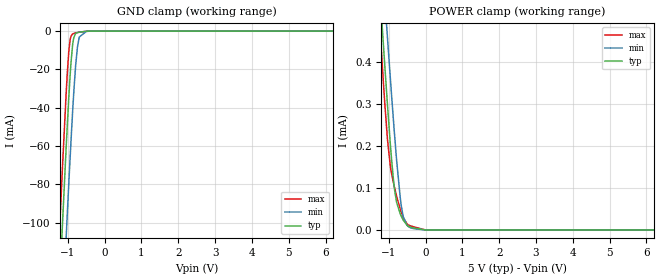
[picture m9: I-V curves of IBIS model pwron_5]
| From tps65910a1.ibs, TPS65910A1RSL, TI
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|   pwron_5 Model
[Model]   pwron_5
Model_type   Input
Vinl = 1.5
Vinh = 3.5
|   typ   min   max
|   (nom PVT)   (fast PVT)   (slow PVT)
C_comp   1.531e-13   1.517e-13   1.557e-13
[Model spec]
|subparameter
Vinl   1.5   1.35   1.65
Vinh   3.5   3.15   3.85
| Where nom  PVT is Nominal Process, 5V, 27C
|   Fast PVT is Strong Process,  5.5V, -40C
|   Slow PVT is Weak Process,   4.5V, 125C
[Voltage Range]   5   4.5   5.5
|Junction Temperature
[Temperature Range]   27   125   -40
[Power Clamp Reference]   5   4.5   5.5
[GND Clamp Reference]   0   0   0
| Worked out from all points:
|   GND clamp passes 1 mA (typ) near -0.76 V on its own axis
|   POWER clamp passes 1 mA (typ) near -1.55 V on its own axis
[GND Clamp]
|   Voltage   I(typ)   I(min)   I(max)
-5V       -1.844A    -1.883A    -1.823A
-1.293V   -163.1mA   -210.9mA   -133.4mA
-1.179V   -115.1mA   -162.9mA   -85.31mA
-1.14V    -98.74mA   -146.5mA   -69.1mA
-1.04V    -58.96mA   -105.7mA   -30.79mA
-974mV    -34.98mA   -79.87mA   -10.93mA
-936.5mV  -22.95mA   -65.75mA   -4.47mA
-855.5mV  -5.262mA   -37.53mA   -1.342mA
-785mV    -1.26mA    -17.51mA   -959.4uA
-689mV    -571.5uA   -3.136mA   -579.6uA
-500mV    -112.8uA   -189uA     -102.9uA
10V       0A         0A         0A
[POWER Clamp]
|   Voltage   I(typ)   I(min)   I(max)
-5V       7.291mA    7.268mA    8.106mA
-1.315V   671.8uA    818.8uA    592.7uA
-1.145V   441.2uA    598uA      351.6uA
-1.105V   389.2uA    547.5uA    299.7uA
-1.034V   299uA      458.5uA    216.8uA
-957.5mV  206.5uA    363.4uA    153.3uA
-840mV    95.24uA    225.5uA    100.2uA
-783.5mV  65.47uA    164.6uA    79.85uA
-655mV    32.02uA    55.69uA    40.94uA
-500mV    11.17uA    11.06uA    14.37uA
-396.5mV  6.491uA    4.97uA     9.483uA
10V       0A         0A         0A
